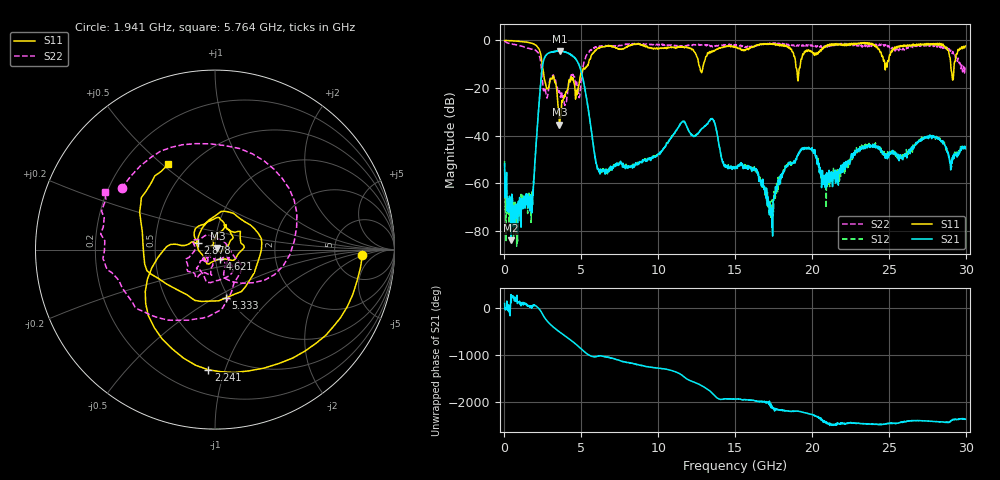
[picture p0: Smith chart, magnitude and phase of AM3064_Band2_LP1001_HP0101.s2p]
# Hz S DB R 50.0
!freq dBS11 angS11 dBS21 angS21 dBS12 angS12 dBS22 angS22
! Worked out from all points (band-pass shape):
!   1600 points, 10 MHz to 29.98 GHz, reference 50 ohm
!   highest |S21| = -4.39 dB at 3.59 GHz (marker M1); lowest = -83.8 dB at 422.4 MHz (marker M2)
!   |S21| within 3 dB of the highest: 2.603 GHz to 4.576 GHz (1.973 GHz wide, 55 % of centre)
!   lowest |S11| = -35.4 dB at 3.571 GHz (marker M3), VSWR 1.03, Z = 51.4 + j1 ohm
!   |S11| at or under -10 dB: 2.45 GHz to 5.453 GHz (3.002 GHz wide, 76 % of centre); 12.64 GHz to 12.95 GHz (312.5 MHz wide, 2.44 % of centre); 18.94 GHz to 19.25 GHz (305.4 MHz wide, 1.6 % of centre)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
!   |S22| runs from -27.3 to -0.3 dB; largest |S21 - S12| = 0.015
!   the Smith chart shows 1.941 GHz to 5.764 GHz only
!   S11 on the Smith chart (normalised r, x): 1.941 GHz: 10, -2; 2.241 GHz: 0.36, -0.88; 2.878 GHz: 0.82, +0.06; 4.621 GHz: 1.05, -0.11; 5.333 GHz: 0.96, -0.56; 5.764 GHz: 0.39, +0.52
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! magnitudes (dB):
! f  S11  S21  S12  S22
! 10 MHz  0.0  -51.8  -50.6  -0.3
! 422.4 MHz  -0.1  -83.8  -69.7  -1.4
! 1.697 GHz  -1.1  -64.7  -67.8  -3.6
! 1.941 GHz  -1.7  -55.8  -56.3  -4.1
! 2.241 GHz  -3.5  -27.2  -27.2  -5.7
! 2.878 GHz  -19.8  -5.3  -5.2  -20.0
! 3.571 GHz  -35.4  -4.5  -4.5  -21.1
! 3.59 GHz  -35.4  -4.4  -4.5  -21.8
! 4.621 GHz  -24.7  -7.7  -7.6  -18.9
! 5.015 GHz  -13.0  -13.7  -13.5  -14.9
! 5.333 GHz  -11.2  -24.0  -23.8  -6.3
! 5.764 GHz  -5.3  -43.2  -43.1  -3.2
! 6.214 GHz  -3.0  -56.0  -56.1  -2.4
! 10 GHz  -3.4  -47.7  -47.9  -1.8
! 13.49 GHz  -4.5  -32.9  -32.9  -2.3
! 15 GHz  -2.6  -53.8  -52.8  -1.9
! 16.37 GHz  -2.0  -53.8  -54.1  -2.4
! 17.31 GHz  -1.6  -69.1  -72.1  -1.4
! 19.99 GHz  -4.6  -45.9  -45.9  -1.9
! 20.83 GHz  -3.0  -61.4  -58.4  -2.4
! 25 GHz  -8.1  -47.5  -47.0  -2.3
! 29.98 GHz  -2.4  -45.4  -44.8  -10.9
